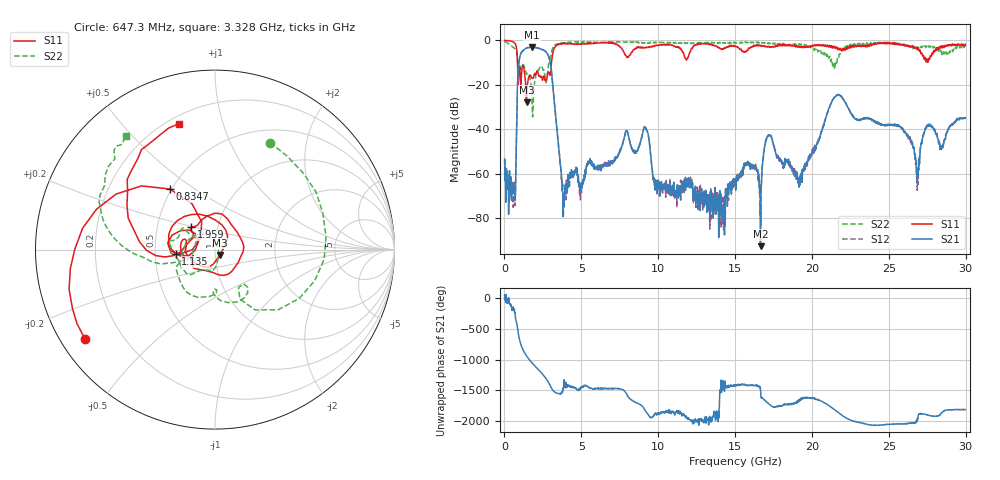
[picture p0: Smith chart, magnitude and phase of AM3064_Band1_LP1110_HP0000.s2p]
# Hz S DB R 50.0
!freq dBS11 angS11 dBS21 angS21 dBS12 angS12 dBS22 angS22
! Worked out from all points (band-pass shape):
!   1600 points, 10 MHz to 29.98 GHz, reference 50 ohm
!   highest |S21| = -3.06 dB at 1.791 GHz (marker M1); lowest = -92.7 dB at 16.65 GHz (marker M2)
!   |S21| within 3 dB of the highest: 1.055 GHz to 2.792 GHz (1.737 GHz wide, 90.3 % of centre)
!   lowest |S11| = -27.9 dB at 1.435 GHz (marker M3), VSWR 1.08, Z = 52.7 - j3.12 ohm
!   |S11| at or under -10 dB: 848.8 MHz to 3.06 GHz (2.211 GHz wide, 113 % of centre)
!   |S22| runs from -34.5 to -0.4 dB; largest |S21 - S12| = 0.0099
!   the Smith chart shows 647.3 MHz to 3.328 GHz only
!   S11 on the Smith chart (normalised r, x): 647.3 MHz: 0.07, -0.31; 834.7 MHz: 0.49, +0.40; 1.135 GHz: 0.64, -0.03; 1.959 GHz: 0.75, +0.19; 3.328 GHz: 0.24, +0.73
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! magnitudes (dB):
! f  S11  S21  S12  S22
! 10 MHz  0.0  -53.5  -53.8  -0.4
! 647.3 MHz  -1.1  -66.7  -67.8  -3.5
! 834.7 MHz  -7.5  -24.9  -24.8  -7.9
! 1.135 GHz  -13.2  -5.1  -5.1  -12.0
! 1.435 GHz  -27.9  -3.5  -3.4  -15.2
! 1.791 GHz  -16.9  -3.1  -3.1  -27.5
! 1.959 GHz  -14.9  -3.2  -3.2  -18.8
! 2.878 GHz  -14.3  -7.3  -7.3  -10.5
! 3.328 GHz  -2.7  -34.0  -33.9  -1.9
! 3.871 GHz  -1.3  -74.0  -74.5  -1.1
! 5.015 GHz  -1.6  -65.3  -68.6  -0.6
! 9.157 GHz  -3.5  -39.0  -39.0  -1.1
! 10 GHz  -2.2  -64.3  -64.2  -0.9
! 15 GHz  -2.7  -63.0  -63.4  -1.2
! 16.65 GHz  -2.5  -92.7  -73.8  -0.9
! 17.2 GHz  -2.6  -43.0  -42.7  -1.1
! 19.11 GHz  -2.5  -64.5  -63.3  -1.8
! 19.99 GHz  -2.8  -50.7  -51.0  -3.0
! 21.64 GHz  -3.4  -24.7  -24.8  -8.7
! 25 GHz  -1.0  -38.2  -37.8  -1.2
! 26.85 GHz  -4.2  -64.2  -67.6  -2.9
! 29.98 GHz  -1.7  -35.1  -34.8  -3.0
